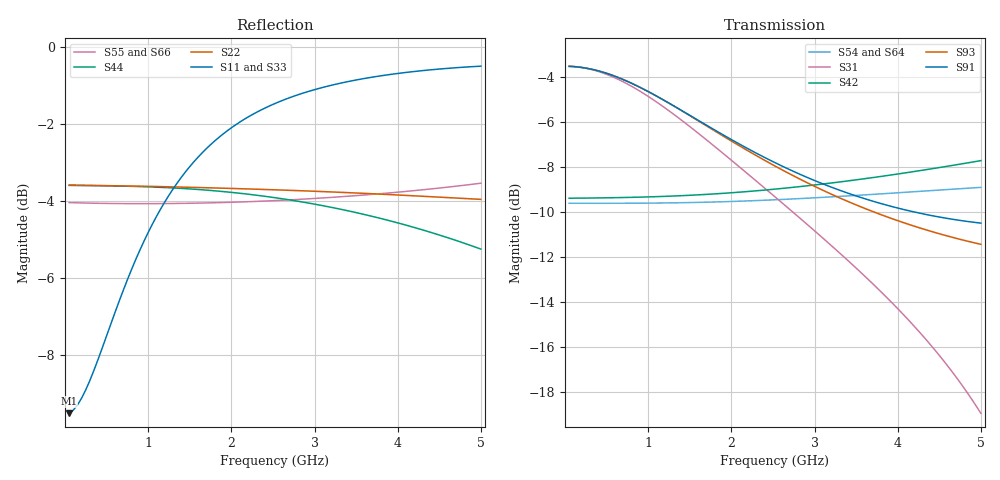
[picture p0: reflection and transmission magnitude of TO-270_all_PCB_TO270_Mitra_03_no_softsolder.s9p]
! Touchstone file from project TO-270_all
! Exported from HFSS 2017.0.0
! Variables:
!  AirBoxH = 25000um
!  AirBoxL = 30000um
!  AirBoxW = 55000um
!  PCB_H = 760um
# GHZ S MA R 50.000000
! Terminal data exported
! Port[1] = 2ED_T
! Port[2] = 3G_Lead_T
! Port[3] = 4D_Lead_T
! Port[4] = 1EG_T
! Port[5] = P_Lead_G1_T1
! Port[6] = P_Lead_G2_T1
! Port[7] = P_Lead_G3_T1
! Port[8] = P_Lead_G4_T1
! Port[9] = P_Lead_D_T1
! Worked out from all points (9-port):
!   100 points, 50 MHz to 5 GHz, reference per port
!   strongest paths, dB at 50 MHz, 1.3 GHz, 2.55 GHz, 3.8 GHz, 5 GHz:
!     S91: -3.5, -5.3, -7.9, -9.6, -10.5
!     S93: -3.5, -5.3, -8.0, -10.1, -11.4
!     S42: -9.4, -9.3, -9.0, -8.4, -7.7
!     S31: -3.5, -5.6, -9.4, -13.6, -19.0
!     S54: -9.6, -9.6, -9.5, -9.2, -8.9
!     S64: -9.6, -9.6, -9.5, -9.2, -8.9
!   lowest |S11| = -9.5 dB at 50 MHz (marker M1), VSWR 2.00
!   |S11| at or under -10 dB: nowhere
